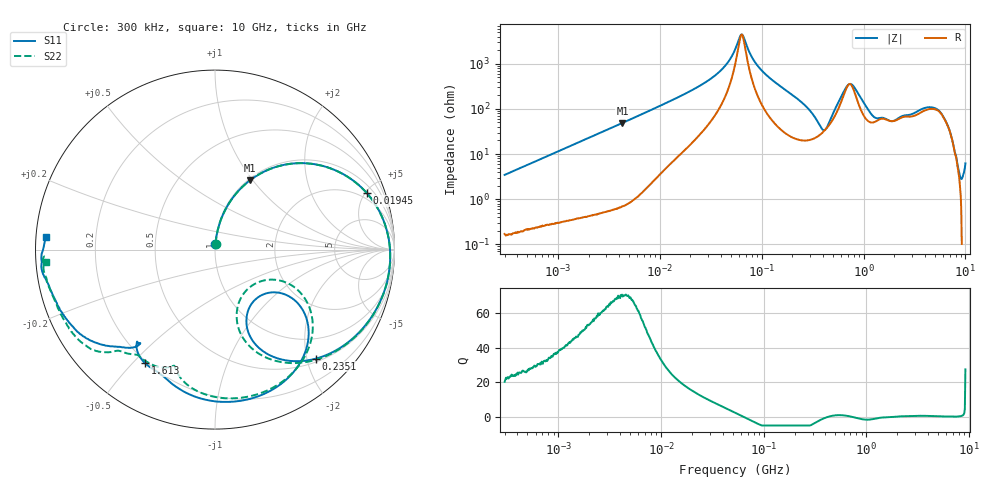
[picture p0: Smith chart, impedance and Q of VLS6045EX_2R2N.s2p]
! S-Parameter Data Generated by TDK Corporation
! Copyright(C) 2019 TDK Corporation.
! All Rights Reserved.
! TDK P/N: VLS6045EX-2R2N (Inductor)
! Property: L=2.2uH at 100kHz
! Size(LxWxT): 6x6x4.5mm
! Model Type: s2p (Touchstone File Format Version 1.0)
! Frequency: DC=Yes Start=0.3MHz Stop=10000MHz 802points Log-sweep
! Model Generated on May 10, 2019
! Port Assignments:
!  1 ---@@@--- 2
! Applicable Conditions:
!  Temperature = 25 degC
!  DC Bias Current = 0 A
!  Small Signal Operation
! Terms and conditions regarding TDK Simulation Models
! (1)This simulation model is being provided solely for informational purposes. Please refer to the specifications of the products in terms of detailed characteristics of such products.
! (2)In no event shall TDK Corporation of any of its subsidiaries be liable for any loss or damage arising, directly or indirectly,
!  From any information contained in this simulation model, including, but not limited to loss or damages arising from any inaccuracies, omissions or errors in connection with such information.
! (3)Any and all copyrights on this simulation model are owned by TDK Corporation.
!  Duplication or redistribution of this simulation model without prior written permission from TDK Corporation is prohibited.
! (4)This simulation model is subject to any modification or change without any prior notice.
! (5)Neither TDK Corporation nor any of its subsidiaries shall make any warranty, express or implied,
!  Including but not limited to the correctness, implied warranties of merchantability and fitness for a particular purpose with respect to this simulation models.
! (6)The use of this simulation model shall be deemed to have consented to the terms and conditions hereof.
# Hz S MA R 50
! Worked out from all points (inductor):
!   801 points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, 300 kHz to 10 GHz, reference 50 ohm
!   read as one part in series: L = 1.83 uH near 318.3 kHz
!   highest Q = 70.4 at 4.301 MHz (marker M1), where L = 1.8 uH
!   self-resonance near 63.74 MHz
!   S11 on the Smith chart (normalised r, x): 300 kHz: 1.00, +0.07; 19.45 MHz: 1.50, +5.12; 235.1 MHz: 0.56, -2.17; 1.613 GHz: 0.19, -0.54; 10 GHz: 0.03, +0.04
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300000  0.03347 85.3  0.9977 -2.0  0.9978 -2.0  0.03334 84.8
1713600  0.1886 77.8  0.9783 -11.0  0.9783 -11.0  0.1886 77.8
4301371  0.4338 63.1  0.8949 -26.1  0.8948 -26.1  0.4338 63.1
9671944  0.7338 40.3  0.6584 -48.0  0.6583 -48.0  0.7338 40.3
1.945436e7  0.9025 20.5  0.3769 -65.9  0.3768 -65.9  0.9026 20.4
3.773551e7  0.9655 5.5  0.1522 -75.9  0.1522 -75.9  0.9656 5.4
5.477226e7  0.977 -2.1  0.04797 -64.9  0.04797 -64.9  0.977 -2.3
6.481723e7  0.9779 -5.7  0.02245 6.4  0.02246 6.4  0.9779 -5.9
1.050124e8  0.9652 -17.2  0.1492 63.4  0.1492 63.4  0.965 -17.6
2.351426e8  0.8287 -47.1  0.4707 35.3  0.4707 35.3  0.8255 -48.5
3.126428e8  0.6706 -62.1  0.6202 14.4  0.6201 14.4  0.6596 -65.1
4.508285e8  0.358 -47.8  0.6782 -31.6  0.6781 -31.6  0.2853 -48.1
5.225392e8  0.5039 -32.2  0.5399 -54.2  0.5398 -54.2  0.4481 -24.8
6.490631e8  0.761 -48.7  0.2553 -67.6  0.2551 -67.6  0.7345 -43.1
7.497801e8  0.834 -63.9  0.1711 -42.1  0.171 -42.1  0.8164 -59.3
9.216398e8  0.8528 -83.9  0.2501 -19.7  0.25 -19.6  0.8375 -80.7
1.180962e9  0.8012 -104.4  0.3558 -36.7  0.3558 -36.6  0.7608 -102.6
1.613252e9  0.7429 -121.7  0.3195 -67.5  0.3197 -67.5  0.7154 -113.3
1.767019e9  0.7178 -126.8  0.3142 -74.5  0.3146 -74.5  0.7302 -118.3
3.932853e9  0.8712 -145.5  0.0885 -150.0  0.08846 -150.2  0.887 -141.4
7.763894e9  0.9726 -174.3  0.02798 -149.8  0.02806 -149.6  0.9607 -172.6
1e10  0.9456 175.7  0.03194 -136.8  0.0318 -137.3  0.946 -175.9
